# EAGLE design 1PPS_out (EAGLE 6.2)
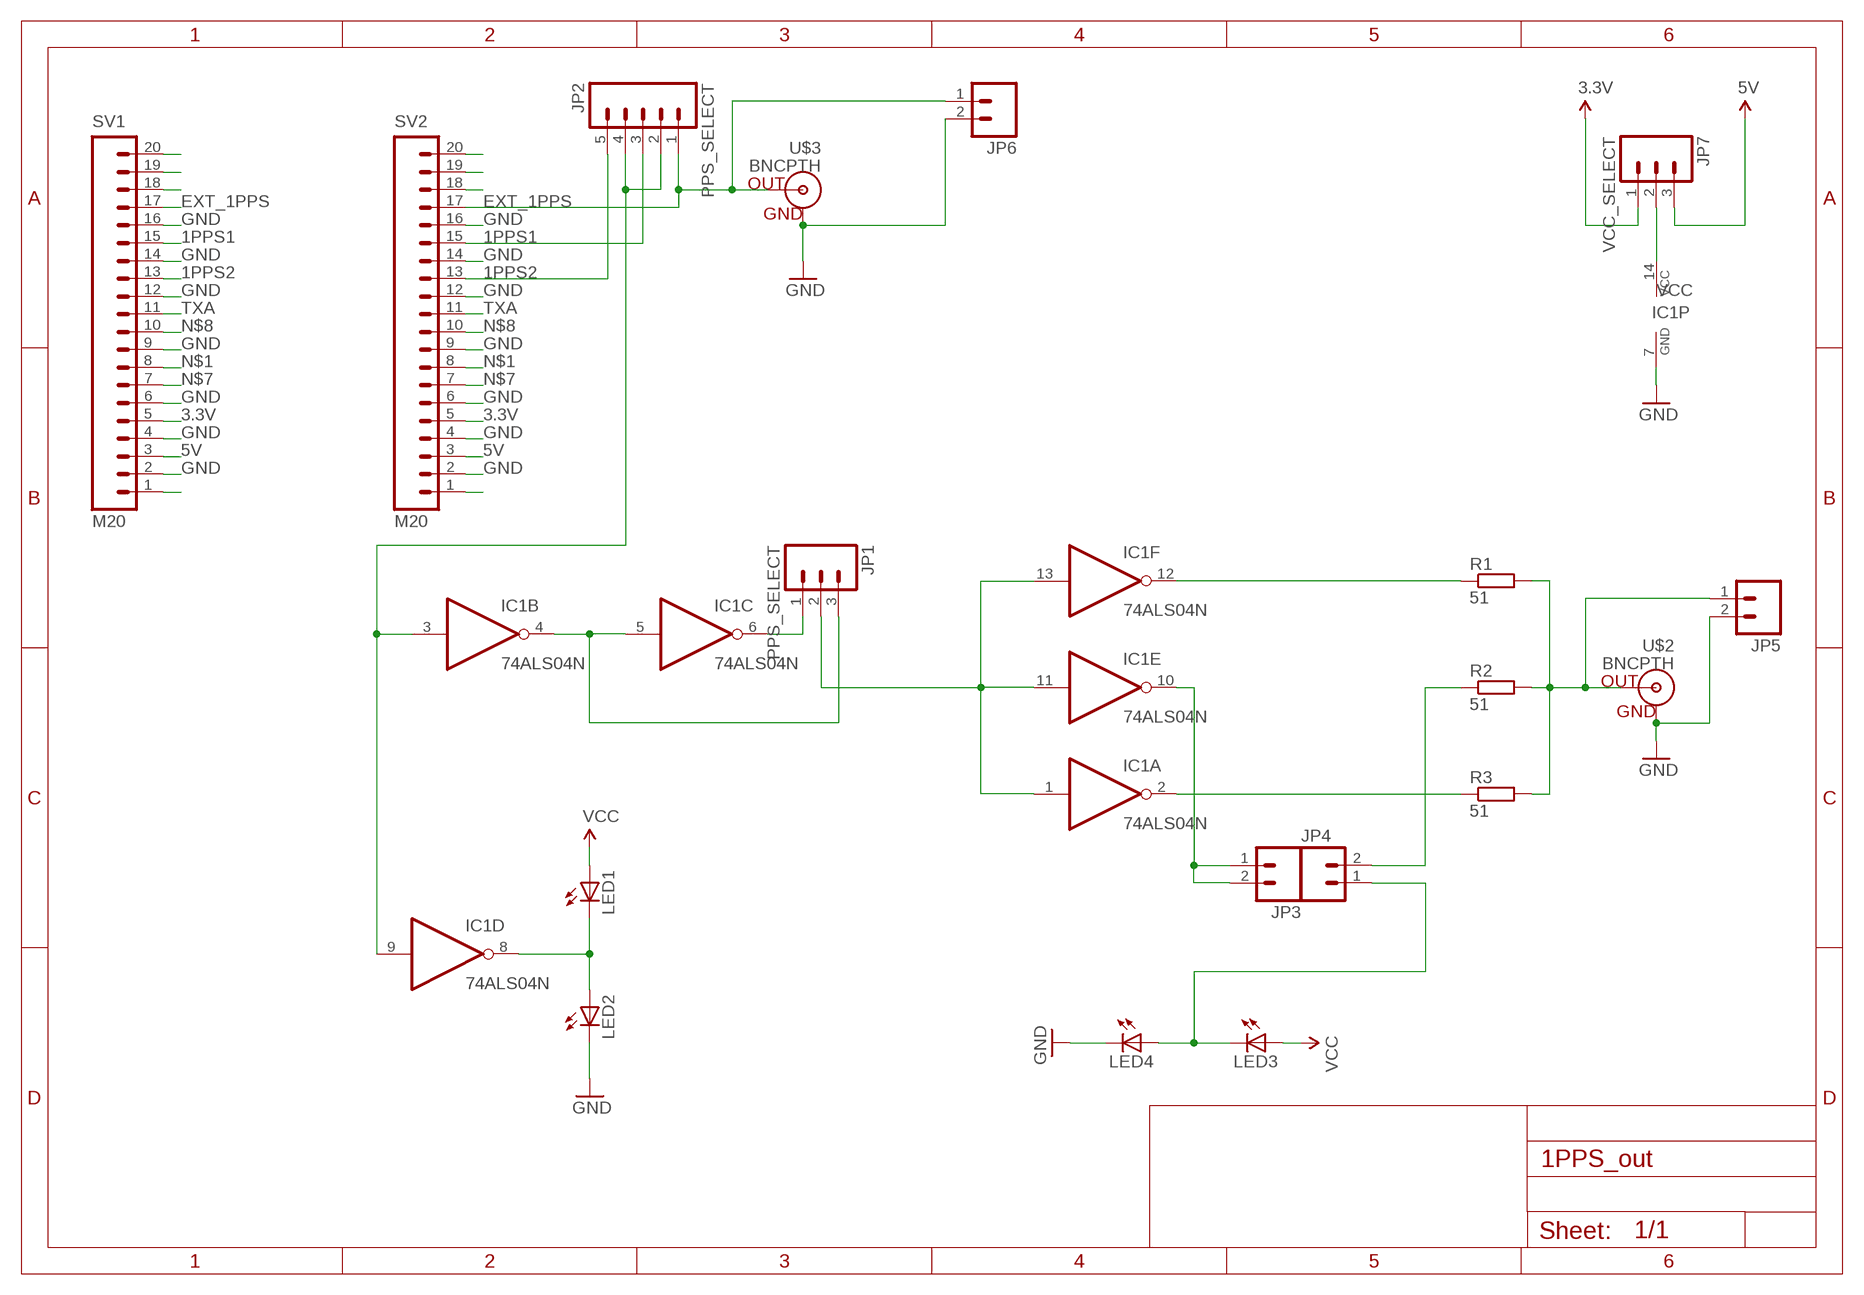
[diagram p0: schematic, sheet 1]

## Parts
IC1  74ALS04N  [DIL14]
JP1  PPS_SELECT  M03LONGPADS  [1X03_LONGPADS]
JP2  PPS_SELECT  M05PTH_LONGPADS  [1X05_LONGPADS]
JP3  M02PTH  [1X02]
JP4  M02PTH  [1X02]
JP5  M02PTH3  [1X02_LONGPADS]
JP6  M02PTH3  [1X02_LONGPADS]
JP7  VСС_SELECT  M03LONGPADS  [1X03_LONGPADS]
LED1  LED5MM  [LED5MM]
LED2  LED5MM  [LED5MM]
LED3  LED5MM  [LED5MM]
LED4  LED5MM  [LED5MM]
R1  51  R-EU_0204/7  [0204/7]
R2  51  R-EU_0204/7  [0204/7]
R3  51  R-EU_0204/7  [0204/7]
SV1  M20  [1X20]
SV2  M20  [1X20]
U$2  BNCPTH  [BNC]
U$3  BNCPTH  [BNC]

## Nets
1PPS: IC1.3(B:I) IC1.9(D:I) JP2.2 JP2.4
1PPS1: JP2.3 SV1.15 SV2.15
1PPS2: JP2.5 SV1.13 SV2.13
3.3V: JP7.1 SV1.5 SV2.5
5V: JP7.3 SV1.3 SV2.3
EXT_1PPS: JP2.1 JP6.1 SV1.17 SV2.17 U$3.S(OUT)
GND: IC1.7(P:GND) JP5.2 JP6.2 LED2.K(C) LED4.K(C) SV1.2 SV1.4 SV1.6 SV1.9 SV1.12 SV1.14 SV1.16 SV2.2 SV2.4 SV2.6 SV2.9 SV2.12 SV2.14 SV2.16 U$2.GND U$3.GND
N$1: SV1.8 SV2.8
N$2: SV2.1
N$3: SV1.1
N$4: SV2.18
N$5: SV2.19
N$6: SV2.20
N$7: SV1.7 SV2.7
N$8: SV1.10 SV2.10
N$9: IC1.12(F:O) R1.1
N$10: IC1.10(E:O) JP3.1 JP3.2
N$11: IC1.2(A:O) R3.1
N$12: JP5.1 R1.2 R2.2 R3.2 U$2.S(OUT)
N$13: IC1.1(A:I) IC1.11(E:I) IC1.13(F:I) JP1.2
N$14: IC1.4(B:O) IC1.5(C:I) JP1.3
N$15: IC1.6(C:O) JP1.1
N$16: IC1.8(D:O) LED1.K(C) LED2.A
N$17: JP4.1 LED3.K(C) LED4.A
N$18: JP4.2 R2.1
N$19: SV1.18
N$20: SV1.19
N$21: SV1.20
TXA: SV1.11 SV2.11
VCC: IC1.14(P:VCC) JP7.2 LED1.A LED3.A

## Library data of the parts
IC1 = 74xx-eu:74*04: Hex INVERTER
JP1 JP7 = SparkFun:M03: Header 3 Standard 3-pin 0.1" header. Use with straight break away headers (SKU : PRT-00116), right angle break away headers (PRT-00553), swiss pins (PRT-00743), machine pins (PRT-00117), and female headers (PRT-00115). Molex polarized connector foot print use with SKU : PRT-08232 with associated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
JP2 = SparkFun:M05: Header 5 Standard 5-pin 0.1" header. Use with straight break away headers (SKU : PRT-00116), right angle break away headers (PRT-00553), swiss pins (PRT-00743), machine pins (PRT-00117), and female headers (PRT-00115). Molex polarized connector foot print use with SKU : PRT-08230 with associated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
JP3-JP6 = SparkFun:M02: Header 2
LED1-LED4 = SparkFun:LED: LEDs
R1-R3 = rcl:R-EU_: RESISTOR, European symbol
SV1 SV2 = SparkFun:M20: This is just like the LOCK variant in that the holes are staggared by 5 mil, but except for the last two holes. They are not altered from the "standard" footprint layout. This is used for a special purpose on the layout of our Graphic LCD Backpack. Make sure you want to use this device before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
U$2 U$3 = SparkFun:BNC: BNC Connector, Mouser Part# 5227161

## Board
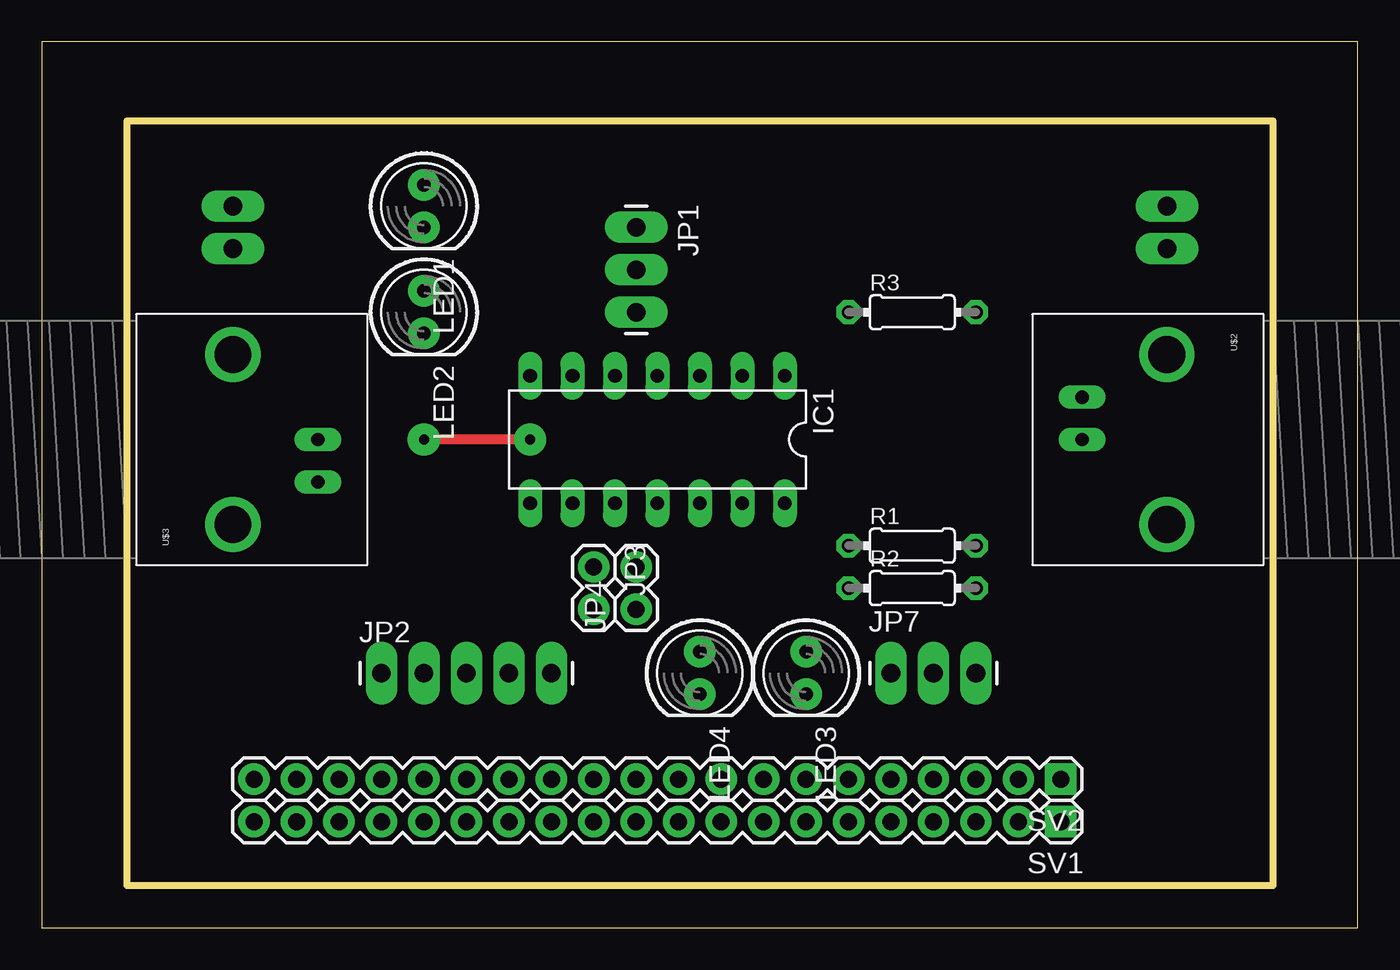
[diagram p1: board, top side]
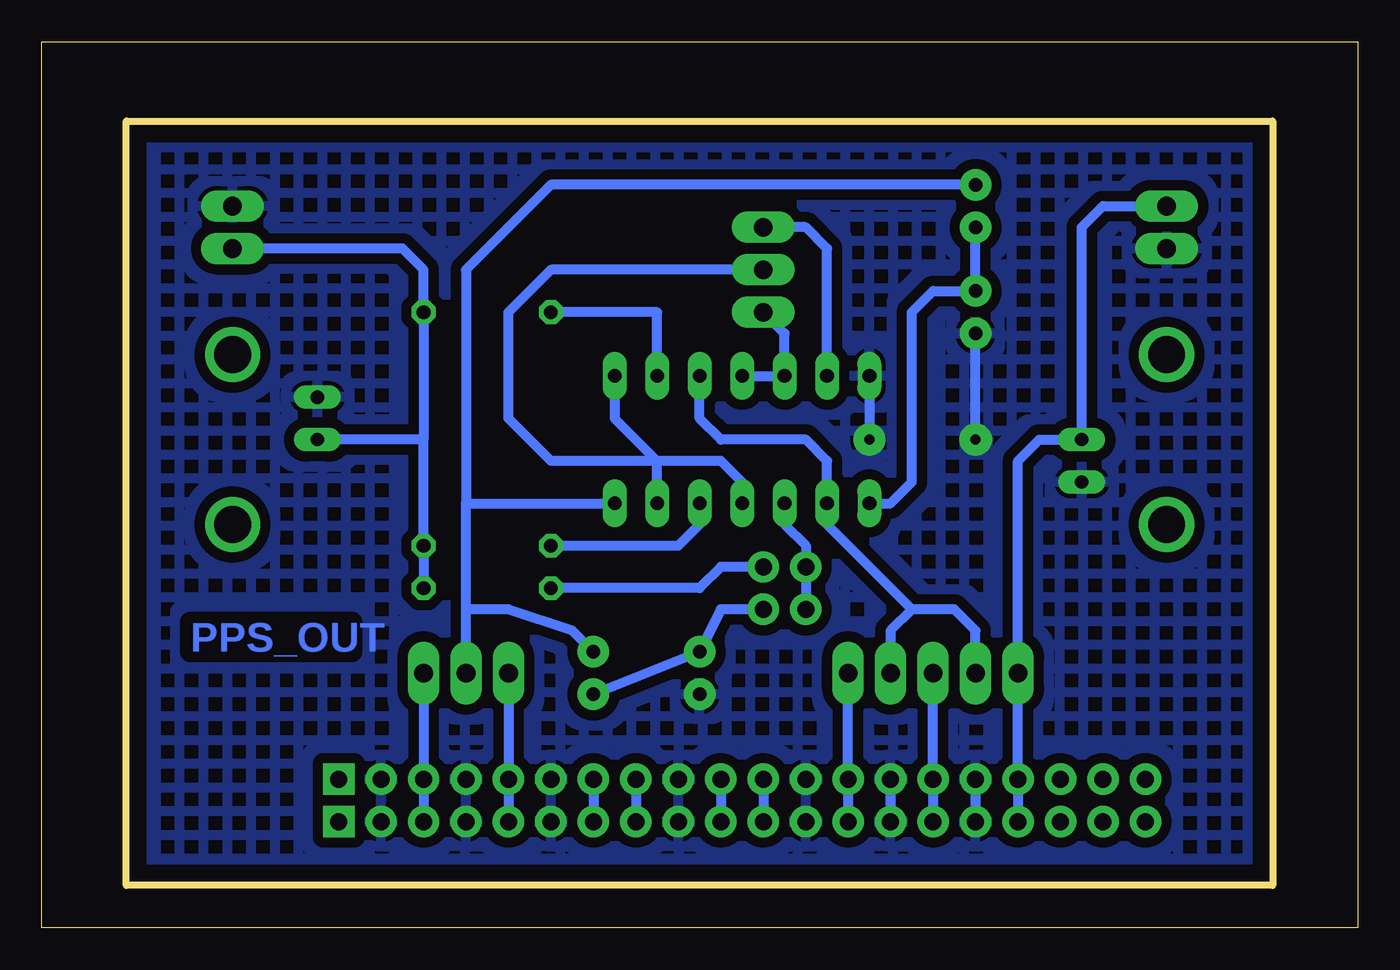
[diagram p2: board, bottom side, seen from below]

Size 78.72 x 53.01 mm. Coordinates in mm from the lower left corner, seen from the top.
Outline: 0,0 78.72,0 78.72,53.01 0,53.01 0,0
Outline: 5.08,2.54 73.66,2.54 73.66,48.26 5.08,48.26 5.08,2.54
Copper layers (1*16): Top 0.035mm / dielectric 1.5mm / Bottom 0.035mm
Design rules: minimum track width 10mil, minimum drill 24mil, track to track 8mil, track to pad 8mil, pad to pad 8mil, via to via 8mil, smd to smd 8mil, copper to edge 40mil, drill to drill 8mil, minimum pad ring 12mil, minimum via ring 12mil, stop-mask expansion 4mil, vias tented up to drill 0mil, thermal gap 10mil

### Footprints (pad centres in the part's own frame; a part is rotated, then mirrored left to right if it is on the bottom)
DIL14 = drill 0.813 long: 1 -7.62,-3.81; 2 -5.08,-3.81; 3 -2.54,-3.81; 4 0,-3.81; 5 2.54,-3.81; 6 5.08,-3.81; 7 7.62,-3.81; 8 7.62,3.81; 9 5.08,3.81; 10 2.54,3.81; 11 0,3.81; 12 -2.54,3.81; 13 -5.08,3.81; 14 -7.62,3.81
1X03_LONGPADS = drill 1.118 pad 1.88 long: 1 0,0; 2 2.54,0; 3 5.08,0
1X05_LONGPADS = drill 1.118 pad 1.88 long: 1 0,0; 2 2.54,0; 3 5.08,0; 4 7.62,0; 5 10.16,0
1X02 = drill 1.016 pad 1.88: 1 0,0; 2 2.54,0
1X02_LONGPADS = drill 1.118 pad 1.88 long: 1 0,0; 2 2.54,0
LED5MM = drill 0.813 pad 1.88: A -1.27,0; K 1.27,0
0204/7 = drill 0.813 octagon: 1 -3.81,0; 2 3.81,0
1X20 = drill 1.016 pad 1.88 square: 1 0,0 | drill 1.016 pad 1.88: 2 2.54,0; 3 5.08,0; 4 7.62,0; 5 10.16,0; 6 12.7,0; 7 15.24,0; 8 17.78,0; 9 20.32,0; 10 22.86,0; 11 25.4,0; 12 27.94,0; 13 30.48,0; 14 33.02,0; 15 35.56,0; 16 38.1,0; 17 40.64,0; 18 43.18,0; 19 45.72,0; 20 48.26,0
BNC = drill 2.2: 3 -5.08,5.08; 4 5.08,5.08 | drill 0.8 long: GND -2.54,0; S 0,0

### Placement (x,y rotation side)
IC1  36.83,29.21 180 top
JP1  35.56,41.91 270 top
JP2  20.32,15.24 0 top
JP3  33.02,21.59 270 top
JP4  35.56,19.05 90 top
JP5  67.31,40.64 90 top
JP6  11.43,43.18 270 top
JP7  50.8,15.24 0 top
LED1  22.86,43.18 270 top
LED2  22.86,36.83 270 top
LED3  45.72,15.24 270 top
LED4  39.37,15.24 270 top
R1  52.07,22.86 0 top
R2  52.07,20.32 0 top
R3  52.07,36.83 0 top
SV1  60.96,6.35 180 top
SV2  60.96,8.89 180 top
U$2  62.23,29.21 270 top
U$3  16.51,29.21 90 top

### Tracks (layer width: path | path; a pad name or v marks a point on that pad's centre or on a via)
1PPS
  Bottom 0.61: 26.67,19.05 31.75,24.13 IC1.9 31.75,27.94 33.02,29.21 38.1,29.21 39.37,30.48 IC1.3 | JP2.2 22.86,17.78 24.13,19.05 26.67,19.05 | JP2.4 27.94,17.78 26.67,19.05
1PPS1
  Bottom 0.61: JP2.3 SV2.15 SV1.15
1PPS2
  Bottom 0.61: JP2.5 SV2.13 SV1.13
3.3V
  Bottom 0.61: JP7.1 SV2.5 SV1.5
5V
  Bottom 0.61: JP7.3 SV2.3 SV1.3
EXT_1PPS
  Bottom 0.61: JP6.1 15.24,43.18 16.51,41.91 U$3.S 19.05,29.21 20.32,27.94 JP2.1 SV2.17 SV1.17
GND  (via drill 0.6, 0.6 pad 1.93)
  Top 0.61: v29.21,29.21 v22.86,29.21
  Bottom 0.61: IC1.7 v29.21,29.21 | v22.86,29.21 LED2.K | SV2.16 SV1.16 | SV2.14 SV1.14
  pour Bottom (isolate 0.61, hatched): 5.08,46.99 73.66,46.99 73.66,2.54 5.08,2.54
N$1
  Bottom 0.61: SV2.8 SV1.8
N$7
  Bottom 0.61: SV2.7 SV1.7
N$8
  Bottom 0.61: SV2.10 SV1.10
N$9
  Bottom 0.61: R1.1 40.64,22.86 39.37,24.13 IC1.12
N$10
  Bottom 0.61: IC1.10 34.29,24.13 33.02,22.86 JP3.1 JP3.2
N$11
  Bottom 0.61: IC1.2 41.91,36.83 R3.1
N$12
  Bottom 0.61: 55.88,29.21 R3.2 55.88,39.37 57.15,40.64 JP5.1 | R2.2 R1.2 55.88,29.21 | 55.88,29.21 U$2.S
N$13
  Bottom 0.61: IC1.1 44.45,30.48 41.91,27.94 | IC1.13 41.91,27.94 | IC1.11 36.83,26.67 38.1,27.94 41.91,27.94 | 41.91,27.94 48.26,27.94 50.8,30.48 50.8,36.83 48.26,39.37 JP1.2
N$14
  Bottom 0.61: IC1.4 IC1.5 34.29,35.56 JP1.3
N$15
  Bottom 0.61: IC1.6 31.75,40.64 33.02,41.91 JP1.1
N$16
  Bottom 0.61: LED1.K LED2.A 25.4,38.1 26.67,36.83 26.67,26.67 27.94,25.4 IC1.8
N$17
  Bottom 0.61: JP4.1 38.1,19.05 LED4.A LED3.K
N$18
  Bottom 0.61: JP4.2 36.83,21.59 38.1,21.59 39.37,20.32 R2.1
TXA
  Bottom 0.61: SV2.11 SV1.11
VCC
  Bottom 0.61: JP7.2 53.34,19.05 | 53.34,19.05 53.34,25.4 | LED1.A 48.26,44.45 53.34,39.37 53.34,25.4 | 53.34,25.4 IC1.14 | LED3.A 46.99,17.78 50.8,19.05 53.34,19.05

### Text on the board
Bottom: PPS_OUT
_tNames: C8 | C6 | C5 | C7 | U2 | JP1 | C1 | JP5 | JP6 | X1 | JP2 | JP7 | JP3 | JP4 | SV1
